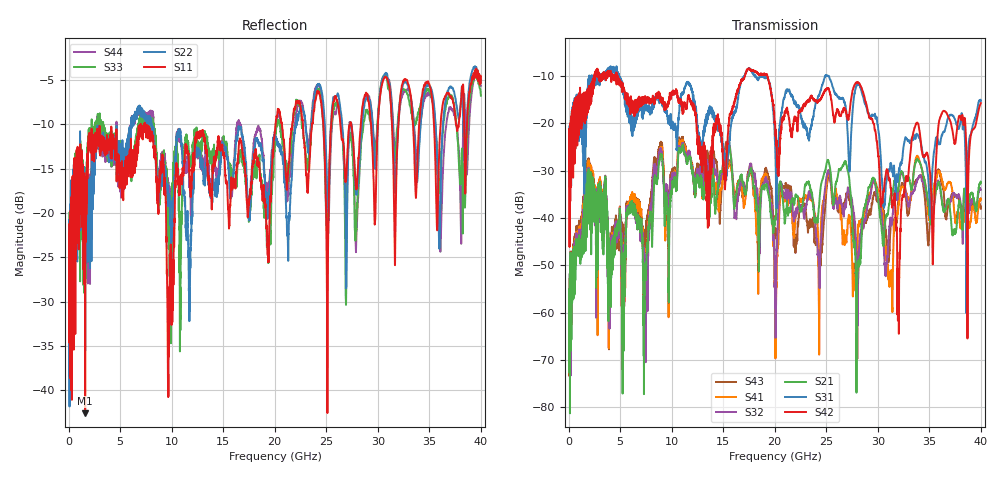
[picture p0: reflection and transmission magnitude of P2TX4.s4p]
!Agilent Technologies,N5245A,MY49151084,A.09.20.08
!Agilent N5245A: A.09.20.08
!Date: Thursday, March 01, 2012 13:54:46
!Correction: S11(Full 4 Port(1,2,3,4))
!S12(Full 4 Port(1,2,3,4))
!S13(Full 4 Port(1,2,3,4))
!S14(Full 4 Port(1,2,3,4))
!S21(Full 4 Port(1,2,3,4))
!S22(Full 4 Port(1,2,3,4))
!S23(Full 4 Port(1,2,3,4))
!S24(Full 4 Port(1,2,3,4))
!S31(Full 4 Port(1,2,3,4))
!S32(Full 4 Port(1,2,3,4))
!S33(Full 4 Port(1,2,3,4))
!S34(Full 4 Port(1,2,3,4))
!S41(Full 4 Port(1,2,3,4))
!S42(Full 4 Port(1,2,3,4))
!S43(Full 4 Port(1,2,3,4))
!S44(Full 4 Port(1,2,3,4))
!S4P File: Measurements: <S11,S12,S13,S14>,
!<S21,S22,S23,S24>,
!<S31,S32,S33,S34>,
!<S41,S42,S43,S44>:
# Hz S  dB  R 50
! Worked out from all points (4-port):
!   3996 points, 50 MHz to 40 GHz, reference 50 ohm
!   strongest paths, dB at 50 MHz, 10.04 GHz, 20.03 GHz, 30.02 GHz, 40 GHz:
!     S42: -25.4, -13.5, -19.9, -26.2, -15.8
!     S31: -24.9, -21.0, -23.9, -20.8, -15.3
!     S21: -57.1, -33.6, -40.3, -35.8, -32.6
!     S32: -57.9, -32.0, -59.1, -35.9, -34.1
!     S41: -56.3, -32.1, -58.2, -34.2, -36.1
!     S43: -58.9, -30.9, -43.5, -36.2, -38.1
!   lowest |S11| = -42.6 dB at 1.61 GHz (marker M1), VSWR 1.01, Z = 50.6 + j0.441 ohm
!   |S11| at or under -10 dB: start of sweep to 7.01 GHz; 7.393 GHz to 20.09 GHz (12.69 GHz wide, 92.4 % of centre); 20.7 GHz to 21.7 GHz (1.005 GHz wide, 4.74 % of centre)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
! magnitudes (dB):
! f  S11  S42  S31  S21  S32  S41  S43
! 50 MHz  -24.4  -25.4  -24.9  -57.1  -57.9  -56.3  -58.9
! 1.61 GHz  -42.6  -17.3  -32.5  -35.2  -33.7  -32.6  -31.3
! 26.8 GHz  -15.5  -17.2  -15.7  -28.0  -37.1  -43.9  -36.7
! 28.08 GHz  -14.8  -11.4  -11.8  -50.2  -54.4  -42.2  -51.8
! 32.02 GHz  -9.6  -54.1  -30.4  -33.3  -33.6  -37.2  -35.7
! 33.67 GHz  -17.9  -20.3  -23.1  -28.3  -32.9  -27.6  -32.2
! 40 GHz  -5.3  -15.8  -15.3  -32.6  -34.1  -36.1  -38.1
